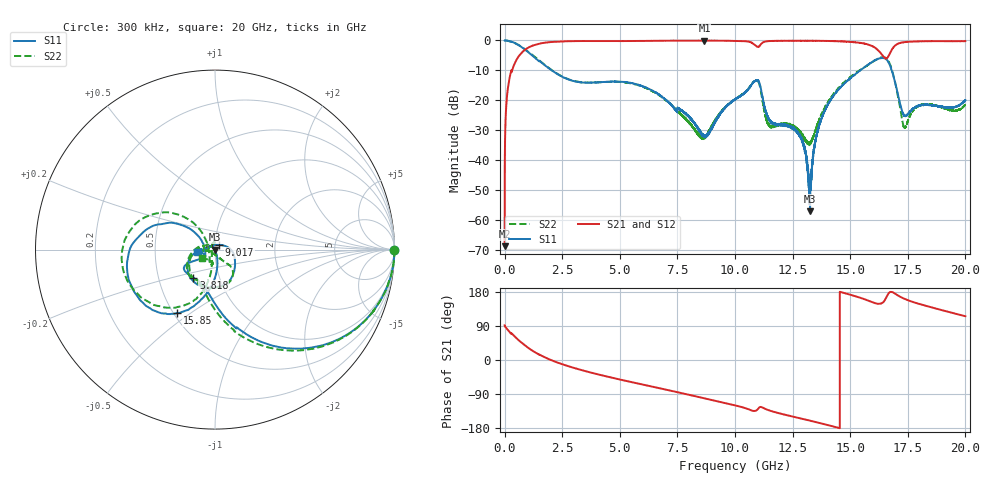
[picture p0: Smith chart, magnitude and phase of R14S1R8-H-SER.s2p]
!{R14S1R8}
!Johanson Technology Inc.
!www.johansontechnology.com
!Test Board Conditions:
!Substrate Type  RO4350B
!Substrate Thickness  20 mil
!Substrate Dk  3.66
!TL Type: GCPW
!TL Trace Width  36 mil
!TL Gap  12 mil
!Electrode orientation  Horizontal
!DUT TOPOLOGY	SERIES
!Mounting Pad LxW  26x36 mil
! Created Wed Nov 25 17:33:21 2020
! 2 Port Network Data from SP1.SP block
! freq  magS11  angS11  magS21  angS21  magS12  angS12  magS22  angS22
# khz S ma R 50
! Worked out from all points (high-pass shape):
!   20001 points, 300 kHz to 20 GHz, reference 50 ohm
!   highest |S21| = -0.04 dB at 8.671 GHz (marker M1); lowest = -68.8 dB at 300 kHz (marker M2)
!   |S21| within 3 dB of the highest: 896.7 MHz to 16.18 GHz (15.28 GHz wide, 179 % of centre); 16.81 GHz to end of sweep
!   lowest |S11| = -57.1 dB at 13.26 GHz (marker M3), VSWR 1.00, Z = 49.9 - j0.0615 ohm
!   |S11| at or under -10 dB: 2.046 GHz to 15.44 GHz (13.39 GHz wide, 153 % of centre); 15.44005 GHz to 15.44186 GHz (1.81 MHz wide, 0.0117 % of centre); 16.8 GHz to end of sweep
!   |S22| runs from -35.0 to 0.0 dB; largest |S21 - S12| = 0.014
!   S11 on the Smith chart (normalised r, x): 300 kHz: open; 3.818 GHz: 0.75, -0.25; 9.017 GHz: 1.05, +0.05; 15.85 GHz: 0.52, -0.45; 20 GHz: 0.82, -0.03
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300  0.9955 -0.0  0.0003636 91.5  0.0002412 84.3  0.9966 -0.1
130300  0.9886 -9.5  0.1456 80.2  0.1462 80.2  0.9885 -9.5
493300  0.8858 -31.3  0.4577 58.9  0.4587 58.9  0.8876 -31.3
1634300  0.4167 -78.2  0.9026 10.4  0.9039 10.4  0.4234 -80.5
3334300  0.1991 -116.6  0.9773 -26.4  0.9774 -26.5  0.2002 -114.9
3818300  0.1974 -127.4  0.9786 -34.3  0.979 -34.3  0.1973 -120.3
6667300  0.1268 -151.1  0.9871 -73.7  0.988 -73.8  0.125 -174.9
8671300  0.02489 107.6  0.9952 -101.0  0.9932 -101.0  0.02327 -111.2
9017300  0.03473 48.4  0.9912 -105.8  0.9922 -105.8  0.03881 -72.5
1.00003e7  0.103 -10.8  0.9856 -119.6  0.9849 -119.6  0.104 -49.0
1.09953e7  0.2165 -119.4  0.7777 -129.5  0.7788 -129.5  0.212 -115.7
1.14873e7  0.04707 -177.7  0.9768 -133.0  0.9753 -133.1  0.03842 120.1
1.27873e7  0.02578 141.2  0.9879 -153.2  0.9872 -153.4  0.0313 122.8
1.32593e7  0.001393 -153.7  0.9856 -160.2  0.9884 -160.1  0.01834 -168.1
1.33343e7  0.007148 -80.5  0.9859 -161.3  0.988 -161.3  0.02078 -151.9
1.35613e7  0.02801 -71.5  0.9864 -164.7  0.9859 -164.5  0.03828 -117.5
1.40213e7  0.0825 -80.5  0.9799 -171.6  0.9819 -171.6  0.09156 -101.1
1.58493e7  0.4114 -120.6  0.839 155.2  0.8404 155.2  0.4078 -127.5
1.66673e7  0.4264 169.4  0.5521 176.0  0.5456 176.6  0.4506 159.1
1.73633e7  0.05493 -178.2  0.9385 161.3  0.9381 161.3  0.03443 -171.6
1.80533e7  0.08287 -147.2  0.9675 146.8  0.966 146.8  0.08268 -109.1
2e7  0.09964 -171.2  0.9724 115.4  0.9702 115.6  0.08512 -148.5
